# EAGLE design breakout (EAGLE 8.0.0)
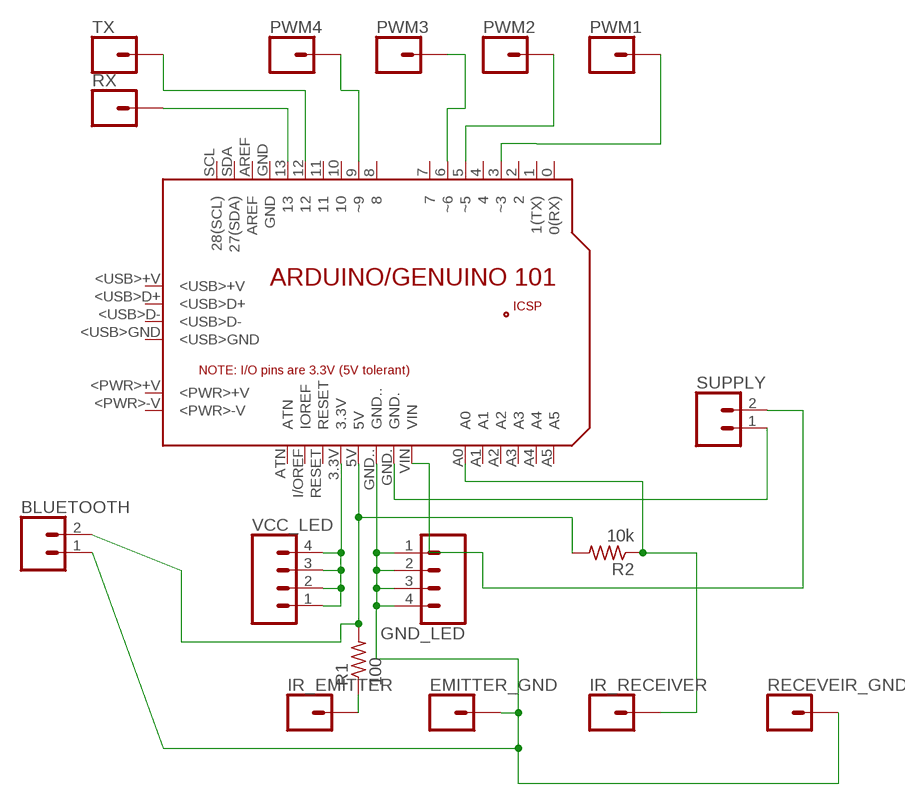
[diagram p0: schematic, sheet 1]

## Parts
BLUETOOTH  CONN_02  [1X02]
EMITTER_GND  CONN_01  [1X01]
GND_LED  CONN_04  [1X04]
IR_EMITTER  CONN_01  [1X01]
IR_RECEIVER  CONN_01  [1X01]
PCB1  ARDUINO_101  [ARDUINO_101]
PWM1  CONN_01  [1X01]
PWM2  CONN_01  [1X01]
PWM3  CONN_01  [1X01]
PWM4  CONN_01  [1X01]
R1  100  RES-US1206  [R1206]
R2  10k  RES-US1206  [R1206]
RECEVEIR_GND  CONN_01  [1X01]
RX  CONN_01  [1X01]
SUPPLY  CONN_02  [1X02]
TX  CONN_01  [1X01]
VCC_LED  CONN_04  [1X04]

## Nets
N$1: PCB1.3.3V VCC_LED.1 VCC_LED.2 VCC_LED.3 VCC_LED.4
N$2: PCB1.GND. SUPPLY.1
N$3: PCB1.3(~3) PWM1.1
N$4: PCB1.9(~9) PWM4.1
N$5: PCB1.5(~5) PWM2.1
N$6: PCB1.6(~6) PWM3.1
N$7: PCB1.VIN SUPPLY.2
N$8: IR_EMITTER.1 R1.1
N$9: PCB1.13 RX.1
N$10: IR_RECEIVER.1 PCB1.A0 R2.1
N$11: PCB1.12 TX.1
N$12: BLUETOOTH.2 PCB1.5V R1.2 R2.2
N$13: BLUETOOTH.1 EMITTER_GND.1 GND_LED.1 GND_LED.2 GND_LED.3 GND_LED.4 PCB1.GND.. RECEVEIR_GND.1
Unconnected: PCB1.0(0(RX)) PCB1.1(1(TX)) PCB1.2 PCB1.4 PCB1.7 PCB1.8 PCB1.10 PCB1.11 PCB1.+5V PCB1.<PWR>+V PCB1.<PWR>-V PCB1.<USB>+V PCB1.<USB>D+ PCB1.<USB>D- PCB1.<USB>GND PCB1.A1 PCB1.A2 PCB1.A3 PCB1.A4 PCB1.A5 PCB1.AREF PCB1.ATN PCB1.GND PCB1.GND_ PCB1.I/OREF(IOREF) PCB1.MISO PCB1.MOSI PCB1.RESET PCB1.RESET. PCB1.SCK PCB1.SCL(28(SCL)) PCB1.SDA(27(SDA))

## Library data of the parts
BLUETOOTH SUPPLY = 03_SparkFun-Connectors:CONN_02: Multi connection point. Often used as Generic Header-pin footprint for 0.1 inch spaced/style header connections
EMITTER_GND IR_EMITTER IR_RECEIVER PWM1-PWM4 RECEVEIR_GND RX TX = 03_SparkFun-Connectors:CONN_01: Single connection point. Often used as Generic Header-pin footprint for 0.1 inch spaced/style header connections
GND_LED VCC_LED = 03_SparkFun-Connectors:CONN_04: Multi connection point. Often used as Generic Header-pin footprint for 0.1 inch spaced/style header connections On any of the 0.1 inch spaced packages, you can populate with these: Break Away Headers - Straight (PRT-00116) Break Away Male Headers - Right Angle (PRT-00553) Female Headers (PRT-00115)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; PROD_ID: CONN-09696
PCB1 = 04_Arduino_Genuino_101:ARDUINO_101: Schematic symbol for representing an Arduino/Genuino 101 board in an EAGLE schematic. Created by Dave Young for Element14. More 101 documentation at: https://www.element14.com/community/docs/DOC-80459/l/intel-genuino-101-development-board More EAGLE documentation at: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
R1 R2 = 00_fab:RES-US: Resistor (US Symbol)

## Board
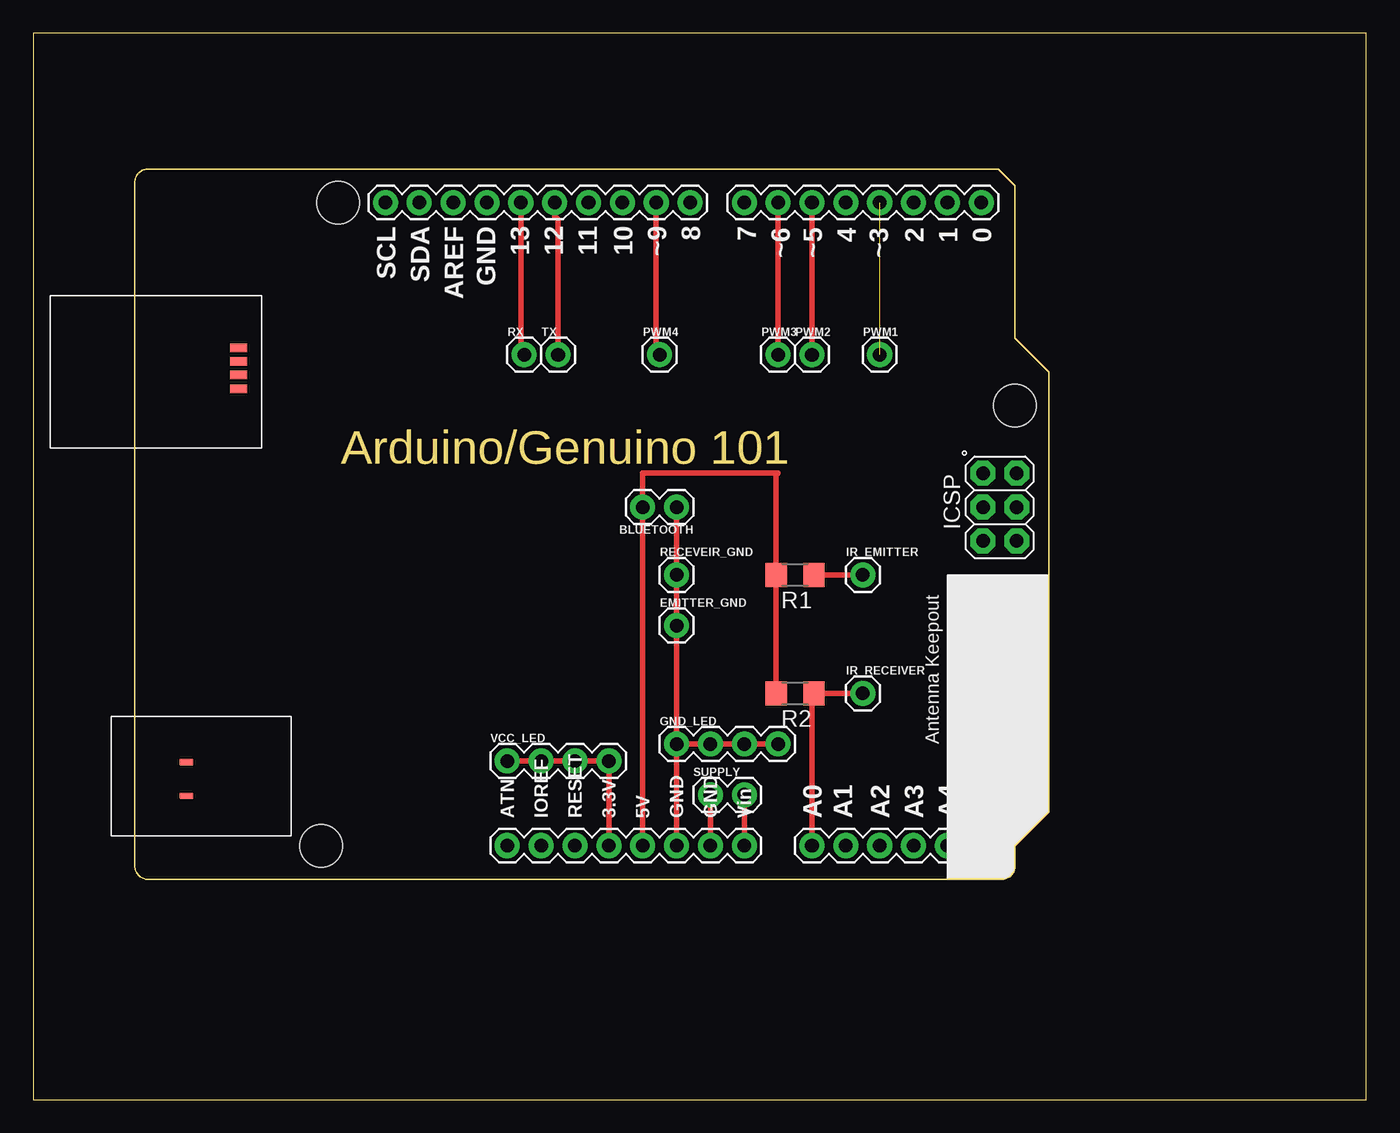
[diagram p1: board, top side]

Size 100 x 80 mm. Coordinates in mm from the lower left corner, seen from the top.
Outline: 0,0 100,0 100,80 0,80 0,0
Copper layers (1*16): Top 0.035mm / dielectric 1.5mm / Bottom 0.035mm
Design rules "default": minimum track width 10mil, minimum drill 24mil, track to track 8mil, track to pad 8mil, pad to pad 8mil, via to via 8mil, smd to smd 8mil, copper to edge 40mil, drill to drill 8mil, minimum pad ring 10mil, minimum via ring 8mil, stop-mask expansion 4mil, vias tented up to drill 0mil, thermal gap 10mil

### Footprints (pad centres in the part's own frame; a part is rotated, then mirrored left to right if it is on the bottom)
1X02 = drill 1.016 pad 1.88: 1 0,0; 2 2.54,0
1X01 = drill 1.016 pad 1.88: 1 0,0
1X04 = drill 1.016 pad 1.88: 1 0,0; 2 2.54,0; 3 5.08,0; 4 7.62,0
ARDUINO_101 = drill 1.016 pad 1.88: 0 27.94,25.4; 1 25.4,25.4; 2 22.86,25.4; 3 20.32,25.4; 3.3V 0,-22.86; 4 17.78,25.4; 5 15.24,25.4; 5V 2.54,-22.86; 6 12.7,25.4; 7 10.16,25.4; 8 6.096,25.4; 9 3.556,25.4; 10 1.016,25.4; 11 -1.524,25.4; 12 -4.064,25.4; 13 -6.604,25.4; A0 15.24,-22.86; A1 17.78,-22.86; A2 20.32,-22.86; A3 22.86,-22.86; A4 25.4,-22.86; A5 27.94,-22.86; AREF -11.684,25.4; ATN -7.62,-22.86; GND -9.144,25.4; GND. 7.62,-22.86; GND.. 5.08,-22.86; I/OREF -5.08,-22.86; RESET -2.54,-22.86; SCL -16.764,25.4; SDA -14.224,25.4; VIN 10.16,-22.86 | drill 1.016 pad 1.88 octagon: +5V 30.607,5.08; GND_ 30.607,0; MISO 28.067,5.08; MOSI 30.607,2.54; RESET. 28.067,0; SCK 28.067,2.54 | smd 1.016 x 0.508: <PWR>+V -31.699,-16.586; <PWR>-V -31.699,-19.126 | smd 1.27 x 0.635: <USB>+V -27.788,14.478; <USB>D+ -27.788,13.487; <USB>D- -27.788,12.471; <USB>GND -27.788,11.43 | hole 3.2: 30.48,-17.78; 30.48,10.16; -20.32,25.4; -21.59,-22.86
R1206 = smd 1.6 x 1.803: 1 -1.422,0; 2 1.422,0

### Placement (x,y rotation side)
BLUETOOTH  48.26,44.45 180 top
EMITTER_GND  48.26,35.56 0 top
GND_LED  48.26,26.67 0 top
IR_EMITTER  62.23,39.37 0 top
IR_RECEIVER  62.23,30.48 0 top
PCB1  43.18,41.91 0 top
PWM1  63.5,55.88 0 top
PWM2  58.42,55.88 0 top
PWM3  55.88,55.88 0 top
PWM4  46.99,55.88 0 top
R1  57.15,39.37 180 top
R2  57.15,30.48 180 top
RECEVEIR_GND  48.26,39.37 0 top
RX  36.83,55.88 0 top
SUPPLY  50.8,22.86 0 top
TX  39.37,55.88 0 top
VCC_LED  35.56,25.4 0 top

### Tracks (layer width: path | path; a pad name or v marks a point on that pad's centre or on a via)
N$1
  Top 0.406: PCB1.3.3V VCC_LED.4 VCC_LED.3 VCC_LED.2 VCC_LED.1
N$2
  Top 0.406: PCB1.GND. SUPPLY.1
N$3  (1 unrouted)
N$4
  Top 0.406: PWM4.1 46.74,55.88 PCB1.9
N$5
  Top 0.406: PWM2.1 PCB1.5
N$6
  Top 0.406: PWM3.1 PCB1.6
N$7
  Top 0.406: PCB1.VIN SUPPLY.2
N$8
  Top 0.406: R1.1 IR_EMITTER.1
N$9
  Top 0.406: RX.1 36.58,56.13 PCB1.13
N$10
  Top 0.406: PCB1.A0 58.42,30.33 R2.1 IR_RECEIVER.1
N$11
  Top 0.406: TX.1 39.37,66.04 39.12,66.29 PCB1.12
N$12
  Top 0.406: R2.2 R1.2 55.73,46.84 55.88,46.99 45.72,46.99 BLUETOOTH.2 PCB1.5V
N$13
  Top 0.406: GND_LED.1 PCB1.GND.. | GND_LED.1 GND_LED.2 GND_LED.3 GND_LED.4 | BLUETOOTH.1 RECEVEIR_GND.1 EMITTER_GND.1 GND_LED.1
